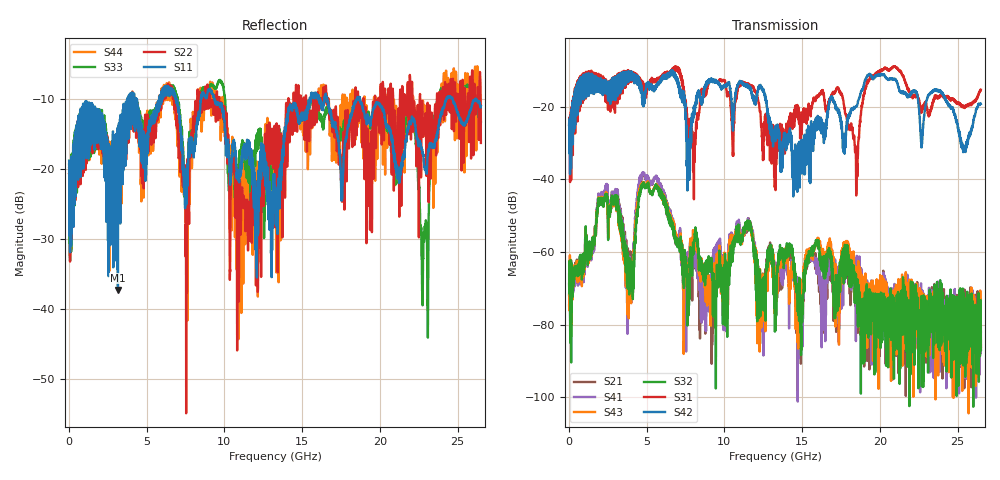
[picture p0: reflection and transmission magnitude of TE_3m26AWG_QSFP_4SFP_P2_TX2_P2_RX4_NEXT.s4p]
!Agilent Technologies,N5222A,MY51421691,A.10.00.00
!Agilent N5222A: A.10.00.00
!Date: Friday, January 30, 2015 12:36:09
!Correction: S11(Full 4 Port(1,2,3,4))
!S12(Full 4 Port(1,2,3,4))
!S13(Full 4 Port(1,2,3,4))
!S14(Full 4 Port(1,2,3,4))
!S21(Full 4 Port(1,2,3,4))
!S22(Full 4 Port(1,2,3,4))
!S23(Full 4 Port(1,2,3,4))
!S24(Full 4 Port(1,2,3,4))
!S31(Full 4 Port(1,2,3,4))
!S32(Full 4 Port(1,2,3,4))
!S33(Full 4 Port(1,2,3,4))
!S34(Full 4 Port(1,2,3,4))
!S41(Full 4 Port(1,2,3,4))
!S42(Full 4 Port(1,2,3,4))
!S43(Full 4 Port(1,2,3,4))
!S44(Full 4 Port(1,2,3,4))
!S4P File: Measurements: <S11,S12,S13,S14>,
!<S21,S22,S23,S24>,
!<S31,S32,S33,S34>,
!<S41,S42,S43,S44>:
# Hz S  dB  R 50.0
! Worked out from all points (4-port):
!   2650 points, 10 MHz to 26.5 GHz, reference 50 ohm
!   strongest paths, dB at 10 MHz, 6.63 GHz, 13.26 GHz, 19.88 GHz, 26.5 GHz:
!     S42: -25.0, -11.1, -25.5, -11.2, -19.2
!     S31: -24.9, -10.2, -30.3, -10.6, -15.3
!     S32: -68.8, -53.2, -72.2, -79.2, -86.9
!     S43: -74.7, -52.7, -68.7, -77.2, -86.2
!     S41: -66.1, -52.1, -69.4, -72.6, -82.0
!     S21: -71.7, -53.0, -75.4, -76.4, -86.9
!   lowest |S11| = -37.3 dB at 3.15 GHz (marker M1), VSWR 1.03, Z = 50.6 - j1.24 ohm
!   |S11| at or under -10 dB: start of sweep to 3.77 GHz; 9.35 GHz to 15.5 GHz (6.146 GHz wide, 49.5 % of centre); 18.72 GHz to 24.29 GHz (5.569 GHz wide, 25.9 % of centre)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
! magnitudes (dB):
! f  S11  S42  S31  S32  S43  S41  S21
! 10 MHz  -18.8  -25.0  -24.9  -68.8  -74.7  -66.1  -71.7
! 3.15 GHz  -37.3  -16.6  -16.9  -46.0  -46.2  -44.0  -43.9
! 3.87 GHz  -14.0  -12.7  -12.8  -61.9  -65.2  -62.4  -60.9
! 4.79 GHz  -14.7  -18.1  -13.6  -41.0  -40.7  -38.3  -38.4
! 8.69 GHz  -9.3  -16.1  -16.9  -64.7  -65.6  -75.5  -72.1
! 11.6 GHz  -17.1  -14.3  -13.9  -52.5  -52.3  -52.2  -51.8
! 26.5 GHz  -11.1  -19.2  -15.3  -86.9  -86.2  -82.0  -86.9
